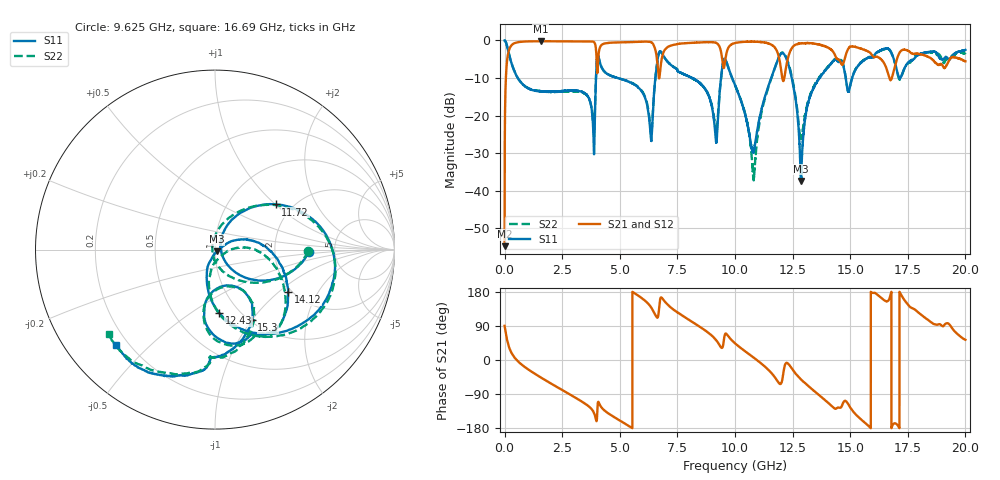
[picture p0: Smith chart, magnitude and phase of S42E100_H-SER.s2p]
! Created Wed Nov 25 21:52:40 2020
# khz S ma R 50
! 2 Port Network Data from SP1.SP block
! freq  magS11  angS11  magS21  angS21  magS12  angS12  magS22  angS22
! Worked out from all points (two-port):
!   20001 points, 300 kHz to 20 GHz, reference 50 ohm
!   highest |S21| = -0.20 dB at 1.57 GHz (marker M1); lowest = -54.8 dB at 300 kHz (marker M2)
!   |S21| within 3 dB of the highest: 162.3 MHz to 3.977 GHz (3.815 GHz wide, 184 % of centre); 6.894 GHz to 9.401 GHz (2.507 GHz wide, 30.8 % of centre)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
!   lowest |S11| = -37.4 dB at 12.86 GHz (marker M3), VSWR 1.03, Z = 51 - j0.917 ohm
!   |S11| at or under -10 dB: 571.9 MHz to 3.968 GHz (3.396 GHz wide, 150 % of centre); 4.912 GHz to 6.543 GHz (1.631 GHz wide, 28.5 % of centre); 9.876 GHz to 11.57 GHz (1.696 GHz wide, 15.8 % of centre)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
!   |S22| runs from -37.2 to 0.0 dB; largest |S21 - S12| = 0.019
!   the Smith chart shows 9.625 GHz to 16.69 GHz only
!   S11 on the Smith chart (normalised r, x): 9.625 GHz: 3.18, -0.14; 11.72 GHz: 1.64, +1.01; 12.43 GHz: 0.81, -0.66; 14.12 GHz: 1.91, -1.16; 15.3 GHz: 1.02, -1.00; 16.69 GHz: 0.16, -0.39
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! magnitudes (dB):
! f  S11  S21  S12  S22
! 300 kHz  0.0  -54.8  -55.1  0.0
! 104.3 MHz  -1.5  -5.5  -5.5  -1.4
! 204.3 MHz  -4.0  -2.3  -2.3  -3.9
! 1.57 GHz  -13.5  -0.2  -0.2  -13.5
! 3.334 GHz  -13.6  -0.2  -0.3  -13.8
! 3.842 GHz  -23.1  -0.3  -0.3  -22.2
! 4.094 GHz  -4.8  -3.0  -3.0  -4.8
! 6.341 GHz  -25.7  -0.4  -0.4  -24.2
! 6.667 GHz  -4.1  -8.3  -8.3  -4.2
! 9.164 GHz  -26.3  -0.6  -0.6  -23.9
! 9.625 GHz  -5.6  -3.5  -3.5  -5.7
! 10 GHz  -11.9  -0.7  -0.7  -11.9
! 10.81 GHz  -29.6  -0.3  -0.3  -37.0
! 11.72 GHz  -7.5  -1.8  -1.8  -7.5
! 12.43 GHz  -9.0  -2.5  -2.4  -8.6
! 12.86 GHz  -37.4  -0.8  -0.8  -26.2
! 13.33 GHz  -13.8  -0.8  -0.8  -13.4
! 14.12 GHz  -6.5  -2.1  -2.1  -6.4
! 15.3 GHz  -7.1  -1.9  -1.8  -7.0
! 16.67 GHz  -2.3  -9.3  -9.5  -2.3
! 16.69 GHz  -2.4  -9.8  -10.1  -2.4
! 20 GHz  -2.5  -5.5  -5.5  -3.3
